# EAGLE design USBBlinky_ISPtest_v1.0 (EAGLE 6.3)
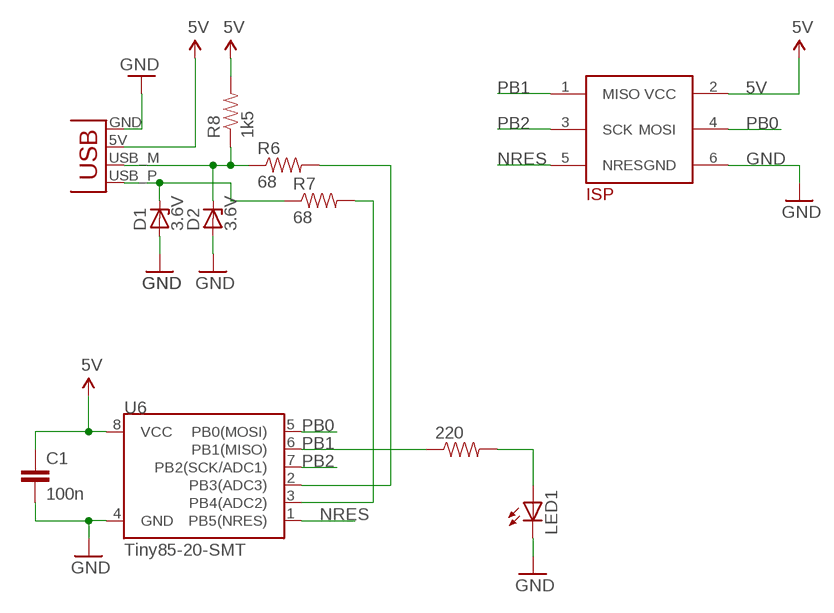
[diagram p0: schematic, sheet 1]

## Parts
220  RESISTOR0805-RES  [0805]
C1  100n  CAP0805  [0805]
D1  3.6V  ZENER-DIODESOD80C  [SOD80C]
D2  3.6V  ZENER-DIODESOD80C  [SOD80C]
JP1  USBPCB  [USB-A-PCB]
LED1  LEDCHIP-LED0805  [CHIP-LED0805]
R6  68  RESISTOR0805-RES  [0805]
R7  68  RESISTOR0805-RES  [0805]
R8  1k5  RESISTOR0805-RES  [0805]
U6  Tiny85-20-SMT  ATTINY45TINY85-20-SMT  [SO08-EIAJ]
U$1  TB_ISPEDGE_2X3  [ISP_EDGE2X3]

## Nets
5V [Power]: C1.1 JP1.5V(VBUS) R8.2 U6.8(VCC) U$1.2(VCC)
GND [Power]: C1.2 D1.A D2.A JP1.GND LED1.C U6.4(GND) U$1.6(GND)
N$1: 220.2 LED1.A
N$5: D2.C JP1.USB_M(D-) R6.1 R8.1
N$6: D1.C JP1.USB_P(D+) R7.1
N$12: R7.2 U6.3(PB4(ADC2))
N$13: R6.2 U6.2(PB3(ADC3))
NRES: U6.1(PB5(NRES)) U$1.5(NRES)
PB0: U6.5(PB0(MOSI)) U$1.4(MOSI)
PB1: 220.1 U6.6(PB1(MISO)) U$1.1(MISO)
PB2: U6.7(PB2(SCK/ADC1)) U$1.3(SCK)

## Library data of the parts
220 = SparkFun-Resistors:RESISTOR: Resistor
C1 = SparkFun-Capacitors:CAP: Capacitor
D1 D2 = diode:ZENER-DIODE: Z-Diode
JP1 = SparkFun-Connectors:USB: USB Connectors USB-B-PTH is fully proven SKU : PRT-00139/CONN-08278 USB-miniB is fully proven SKU : PRT-00587 USB-A-PCB is untested. USB-A-H is throughly reviewed, but untested. Spark Fun Electronics SKU : PRT-00437 USB-B-SMT is throughly reviewed, but untested. Needs silkscreen touching up.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
LED1 = led:LED: LED
R6-R8 = SparkFun-Passives:RESISTOR: Resistor
U6 = SparkFun-DigitalIC:ATTINY45: Atmel 8-pin 2/4/8kB flash uC; PROD_ID: IC-09092
U$1 = tb_custom:TB_ISPEDGE_2X3: AVR-ISP connector an Platinenrand

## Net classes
1 Power: width 0.305 mm, clearance 0.305 mm

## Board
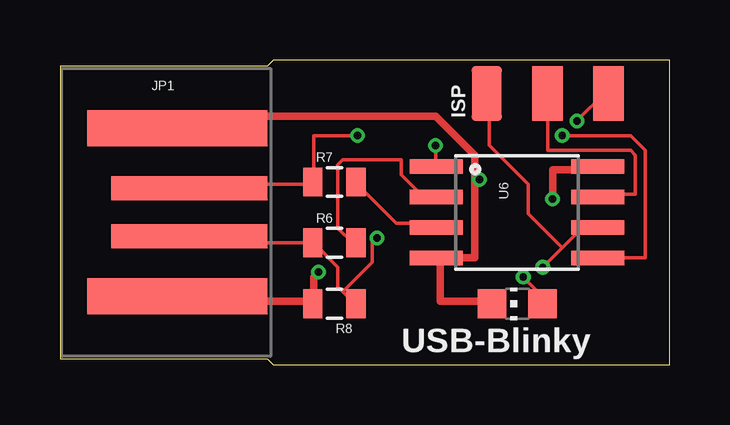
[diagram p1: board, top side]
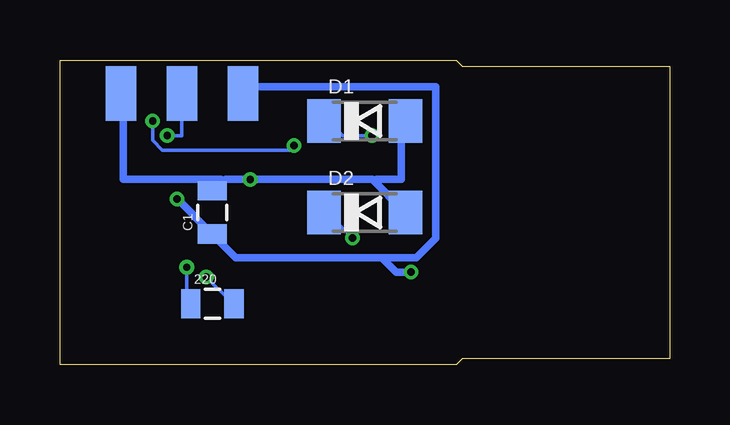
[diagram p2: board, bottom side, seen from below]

Size 25.4 x 12.7 mm. Coordinates in mm from the lower left corner, seen from the top.
Outline: 0,0.25 8.64,0.25 8.89,0 25.4,0 25.4,12.7 8.89,12.7 8.64,12.45 0,12.45 0,0.25
Copper layers (1*16): Top 0.035mm / dielectric 1.5mm / Bottom 0.035mm
Design rules "ITEADstudio_DRC": minimum track width 6mil, minimum drill 12mil, track to track 6mil, track to pad 6mil, pad to pad 6mil, via to via 6mil, smd to smd 0mil, copper to edge 10mil, drill to drill 10mil, minimum pad ring 10mil, minimum via ring 6mil, stop-mask expansion 2mil, vias tented up to drill 100mil, thermal gap 10mil

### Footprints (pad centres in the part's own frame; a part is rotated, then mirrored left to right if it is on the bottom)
0805 = smd 0.8 x 1.2: 1 -0.9,0; 2 0.9,0
SOD80C = smd 1.4 x 1.8: A 1.7,0; C -1.7,0
USB-A-PCB = smd 7.5 x 1.5: 5V -0.2,-3.5; GND -0.2,3.5 | smd 6.5 x 1: USB_M 0.3,-1; USB_P 0.3,1
CHIP-LED0805 = smd 1.2 x 1.2: A 0,-1.05; C 0,1.05
SO08-EIAJ = smd 0.61 x 2.21: 1 -1.905,-3.378; 2 -0.635,-3.378; 3 0.635,-3.378; 4 1.905,-3.378; 5 1.905,3.353; 6 0.635,3.353; 7 -0.635,3.353; 8 -1.905,3.353
ISP_EDGE2X3 = smd 2.286 x 1.27: 1 -0.127,2.54; 3 -0.127,0; 5 -0.127,-2.54 | smd 2.286 x 1.27 bottom: 2 -0.127,2.54; 4 -0.127,0; 6 -0.127,-2.54

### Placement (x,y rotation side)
220  19.05,2.54 0 bottom
C1  19.05,6.35 90 bottom
D1  12.7,10.16 0 bottom
D2  12.7,6.35 0 bottom
JP1  5.08,6.35 0 top
LED1  19.05,2.54 90 top
R6  11.43,5.08 0 top
R7  11.43,7.62 0 top
R8  11.43,2.54 180 top
U6  19.05,6.35 270 top
U$1  20.32,11.43 90 top

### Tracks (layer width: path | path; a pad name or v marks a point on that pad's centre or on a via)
5V  (via drill 0.3)
  Top 0.305: v20.52,6.91 20.52,8.13 22.35,8.13 U6.8 | JP1.5V 5.08,2.85 5.08,2.64 10.36,2.64 R8.2 10.57,2.64 10.57,3.66 v10.77,3.86
  Bottom 0.305: 11.99,4.47 10.57,4.47 9.75,5.28 9.75,11.58 17.48,11.58 17.68,11.38 U$1.2 | 11.99,4.47 18.09,4.47 18.9,5.28 C1.1 19.1,5.49 v20.52,6.91 | 11.99,4.47 11.38,3.86 v10.77,3.86
GND  (via drill 0.3)
  Top 0.305: LED1.C 17.88,2.64 15.85,2.64 15.85,4.27 U6.4 15.85,4.47 17.27,4.47 17.27,7.72 | 17.27,7.72 17.27,8.74 15.65,10.36 5.08,10.36 5.08,9.96 JP1.GND | 17.27,7.72 v17.48,7.72
  Bottom 0.305: 18.59,7.62 18.49,7.72 v17.48,7.72 12.39,7.72 12.29,7.62 | 18.59,7.62 18.9,7.32 C1.2 | 12.29,7.62 11.18,6.5 D2.A | D1.A 11.18,10.16 11.18,7.72 12.19,7.72 12.29,7.62 | U$1.6 22.76,11.18 22.76,7.72 18.69,7.72 18.59,7.62
N$1  (via drill 0.3)
  Top 0.152: v19.3,3.66 19.91,3.05 19.91,2.64 LED1.A
  Bottom 0.152: v19.3,3.66 18.29,2.64 220.2
N$5  (via drill 0.3)
  Top 0.152: 11.79,3.05 11.58,3.25 11.58,4.06 10.57,5.08 R6.1 5.49,5.08 5.49,5.28 JP1.USB_M | 11.79,3.05 12.19,2.64 R8.1 | v13.21,5.28 13.01,5.08 13.01,4.27 11.79,3.05
  Bottom 0.152: v13.21,5.28 14.22,6.3 D2.C
N$6  (via drill 0.3)
  Top 0.152: JP1.USB_P 5.49,7.52 10.36,7.52 R7.1 10.57,7.72 10.57,9.55 v12.39,9.55
  Bottom 0.152: v12.39,9.55 13.61,9.55 14.22,10.16 D1.C
N$12
  Top 0.152: R7.2 12.39,7.52 14.02,5.89 15.65,5.89 U6.3
N$13
  Top 0.152: R6.2 12.19,5.08 11.58,5.69 11.58,8.33 11.79,8.53 14.22,8.53 14.22,7.92 15.04,7.11 15.65,7.11 U6.2
NRES  (via drill 0.3)
  Top 0.152: v15.65,9.14 15.65,8.33 U6.1 | v21.54,10.16 22.76,11.38 U$1.5
  Bottom 0.152: v15.65,9.14 15.85,8.94 21.13,8.94 21.54,9.35 v21.54,10.16
PB0  (via drill 0.3)
  Top 0.152: v20.93,9.55 23.77,9.55 24.38,8.94 24.38,4.47 22.55,4.47 U6.5
  Bottom 0.152: 20.45,10.79 U$1.4 20.32,9.55 v20.93,9.55
PB1  (via drill 0.3)
  Top 0.152: 20.93,4.88 21.74,5.69 22.35,5.69 U6.6 | 20.93,4.88 v20.12,4.06 | 20.93,4.88 19.51,6.3 19.51,7.52 17.88,9.14 17.88,11.18 U$1.1
  Bottom 0.152: v20.12,4.06 20.12,2.64 220.1
PB2
  Top 0.152: U$1.3 20.32,8.94 23.77,8.94 23.98,8.74 23.98,7.11 22.55,7.11 U6.7

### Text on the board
tPlace: ISP | USB-Blinky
